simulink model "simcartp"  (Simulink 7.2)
settings: Solver=ode45  StartTime=0.0  StopTime=500.0  RelTol=1e-3
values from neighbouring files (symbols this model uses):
  A = [0,1,0,0;0,0,-m/M*g,0;0,0,0,1;0,0,g/l*(M+m)/M,0]    [cartp.m]
  B = [0,0;1/M,-1/(l*M);0,0;-1/(M*l),1/l^2*(M+m)/(M*m)]    [cartp.m]
  C = [1,0,0,0;0,0,1,0]    [cartp.m]
  D = zeros(2)    [cartp.m]
  K = Ktot(1:4)    [cartp.m]
  ki = Ktot(5)    [cartp.m]
  L = -place(A',C(1,:)',roots(pobs))'    [cartp.m]
undefined symbols (not defined in the file or in its folder): Reference

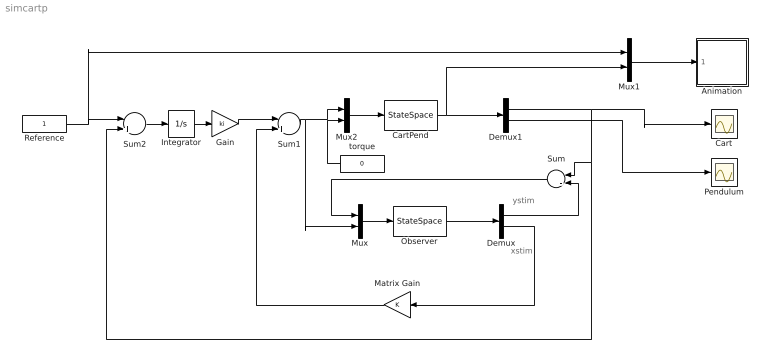
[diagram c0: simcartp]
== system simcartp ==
  note: xstim
  note: ystim
  Animation : Subsystem  mask(Pendulum plot){RefBlock=Reference}
      mask prompts: RefBlock "DC reference signal block name:"
      mask help: Pendulum plot
  Cart : Scope
  CartPend : StateSpace  A=A  B=B  C=C  D=D  X0=[0;0;0.1;0]
  Demux : Demux  Outputs=[1;4]
  Demux1 : Demux  Outputs=2
  Gain : Gain  Gain=ki
  Integrator : Integrator
  Matrix Gain : Gain  Orientation=left  Gain=K  Multiplication=Matrix(K*u)
  Mux : Mux  Inputs=2
  Mux1 : Mux  Inputs=[1;2]
  Mux2 : Mux  Inputs=2
  Observer : StateSpace  A=A  B=[L,B(:,1)]  C=[C(1,:);eye(4)]  D=zeros(5,2)  X0=[0;0;0;0]
  Pendulum : Scope
  Reference : Constant
  Sum : Sum  Orientation=left  Inputs=|-|+
  Sum1 : Sum  Inputs=|++
  Sum2 : Sum  Inputs=|+-
  torque : Constant  Orientation=left  Value=0
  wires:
  Observer/1 -> Demux/1
  Demux/1 -> Sum/2
  Integrator/1 -> Gain/1
  Sum2/1 -> Integrator/1
  Mux/1 -> Observer/1
  Sum/1 -> Mux/1
  Gain/1 -> Sum1/1
  Sum1/1 -> Mux/2, Mux2/1
  Mux2/1 -> CartPend/1
  Mux1/1 -> Animation/1(in_1)
  CartPend/1 -> Mux1/2, Demux1/1
  Reference/1 -> Sum2/1, Mux1/1
  Demux/2 -> Matrix Gain/1
  Matrix Gain/1 -> Sum1/2
  Demux1/1 -> Sum2/2, Sum/1, Cart/1
  Demux1/2 -> Pendulum/1
  torque/1 -> Mux2/2

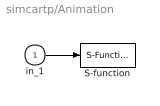
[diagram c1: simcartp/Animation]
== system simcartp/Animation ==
  in_1 : Inport
  S-function : S-Function  FunctionName=pendan  Parameters=RefBlock  EnableBusSupport=off
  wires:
  in_1/1 -> S-function/1
